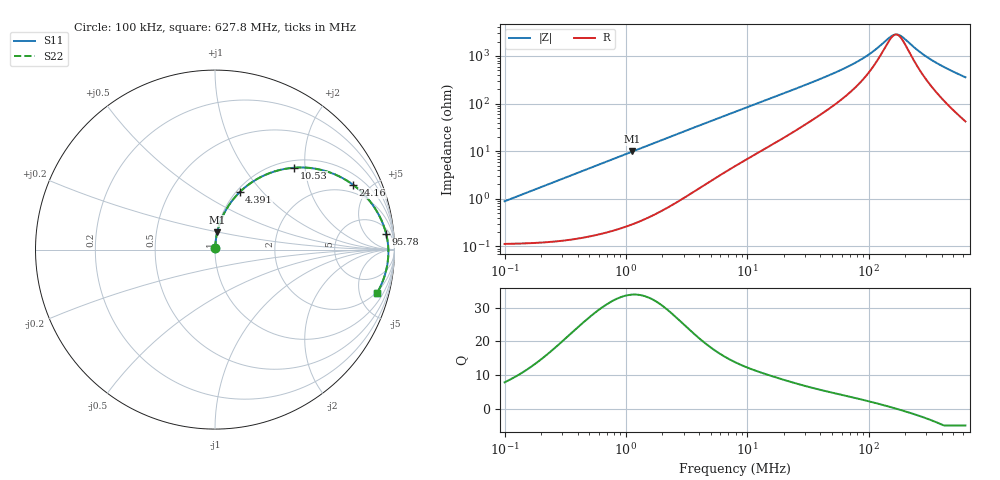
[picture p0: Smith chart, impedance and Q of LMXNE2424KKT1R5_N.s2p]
! LMXNE2424KKT1R5_N  S-PARAMETER MODEL  ( General Type )
! Model Generated by TAIYO YUDEN Corporation (https://www.yuden.co.jp/en/)
! Version 1.0
! TAIYO YUDEN Control No. 191023NI43SB-FBB
! Copyright(c) 2019 TAIYO YUDEN CO.,LTD. All Rights Reserved.
! Product Description (link to TY-COMPAS)
! https://ds.yuden.co.jp/TYCOMPAS/or/detail?pn=LMXNE2424KKT1R5MN&u=M
! Products Name : Inductors
! Characteristics :
!  Inductance : 1.5 uH , SRF(min) : 94 MHz , DC Resistance(max) : 0.132 Ohm
!  Rated Current : Saturation :1550 mA , Temp Rise : 1160 mA (40 degC)
!  Case Size : 2.4 x 2.4 / 0.095 x 0.095 [mm/inch] , Thickness : 1 / 0.039 [mm/inch]
!  (Conditions: Temperature = 25 degC , DC Bias Current/Voltage = 0A / 0V)
! External Node Assignments :
!  1  o---GGG---o  2
! GND o---------o GND
! Frequency Range : 0.1MHz  -  627.813588MHz  [ 402 STEP ]
# MHz S RI R 50
! Freq[MHz].  S11 Real  S11 Imag  S21 Real  S21 Imag  S12 Real  S12 Imag  S22 Real  S22 Imag
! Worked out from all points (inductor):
!   401 points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, 100 kHz to 627.8 MHz, reference 50 ohm
!   read as one part in series: L = 1.4 uH near 104.5 kHz
!   highest Q = 33.8 at 1.132 MHz (marker M1), where L = 1.39 uH
!   self-resonance near 168.1 MHz
!   S11 on the Smith chart (normalised r, x): 100 kHz: 1.00, +0.02; 4.391 MHz: 1.04, +0.75; 10.53 MHz: 1.15, +1.76; 24.16 MHz: 1.51, +3.93; 95.78 MHz: 9, +18; 627.8 MHz: 1.84, -7.09
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0.1  0.0012 0.00877  0.9988 -0.00877  0.9988 -0.00877  0.0012 0.00877
0.43265  0.00293 0.0377  0.9971 -0.0377  0.9971 -0.0377  0.00293 0.0377
1.132134  0.0124 0.0971  0.9876 -0.0971  0.9876 -0.0971  0.0124 0.0971
1.87186  0.0305 0.1567  0.9695 -0.1567  0.9695 -0.1567  0.0305 0.1567
2.962507  0.0698 0.2356  0.9302 -0.2356  0.9302 -0.2356  0.0698 0.2356
4.390983  0.1367 0.3191  0.8633 -0.3191  0.8633 -0.3191  0.1367 0.3191
7.923469  0.3216 0.4322  0.6784 -0.4322  0.6784 -0.4322  0.3216 0.4322
10.52797  0.442 0.4563  0.558 -0.4563  0.558 -0.4563  0.442 0.4563
15.26696  0.6044 0.4409  0.3956 -0.4409  0.3956 -0.4409  0.6044 0.4409
24.16233  0.7687 0.3615  0.2313 -0.3615  0.2313 -0.3615  0.7687 0.3615
34.28088  0.852 0.2832  0.148 -0.2832  0.148 -0.2832  0.852 0.2832
61.85938  0.9286 0.1608  0.0714 -0.1608  0.0714 -0.1608  0.9286 0.1608
95.78491  0.9543 0.0854  0.0457 -0.0854  0.0457 -0.0854  0.9543 0.0854
114.0916  0.96 0.058  0.04 -0.058  0.04 -0.058  0.96 0.058
148.3162  0.9649 0.0185  0.0351 -0.0185  0.0351 -0.0185  0.9649 0.0185
165.448  0.9658 0.00232  0.0342 -0.00232  0.0342 -0.00232  0.9658 0.00232
180.5676  0.966 -0.0107  0.034 0.0107  0.034 0.0107  0.966 -0.0107
197.0689  0.9659 -0.0238  0.0341 0.0238  0.0341 0.0238  0.9659 -0.0238
261.847  0.9624 -0.0682  0.0376 0.0682  0.0376 0.0682  0.9624 -0.0682
325.8318  0.9559 -0.1054  0.0441 0.1054  0.0441 0.1054  0.9559 -0.1054
452.2849  0.9375 -0.1687  0.0625 0.1687  0.0625 0.1687  0.9375 -0.1687
627.8136  0.9026 -0.243  0.0974 0.243  0.0974 0.243  0.9026 -0.243
